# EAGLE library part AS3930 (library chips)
Single Channel Low Frequency Wakeup Receiver
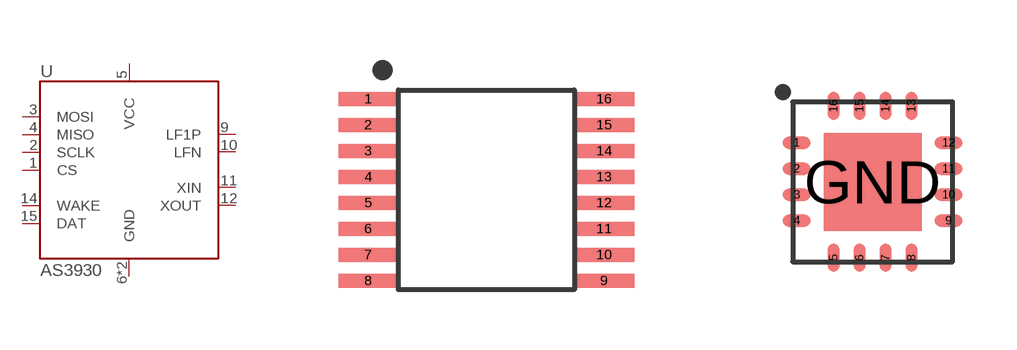
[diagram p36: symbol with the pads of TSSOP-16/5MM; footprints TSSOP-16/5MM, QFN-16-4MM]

Designator prefix U

## AS3930-BTST  [TSSOP-16/5MM]
1  CS
2  SCLK
3  MOSI
4  MISO
5  VCC
6  GND
9  LF1P
10  LFN
11  XIN
12  XOUT
13  GND
14  WAKE
15  DAT

## AS3930-BQFT (DIGIKEY: AS3930-BQFTCT-ND)  [QFN-16-4MM]
3  LF1P
4  LFN
5  XIN
6  XOUT
7  GND
8  WAKE
9  DAT
11  CS
12  SCLK
13  MOSI
14  MISO
15  VCC
16  GND
GND  GND

## Footprint TSSOP-16/5MM (pad centres in mm)
smd 1.5 x 0.35: 1 -2.95,2.275; 2 -2.95,1.625; 3 -2.95,0.975; 4 -2.95,0.325; 5 -2.95,-0.325; 6 -2.95,-0.975; 7 -2.95,-1.625; 8 -2.95,-2.275; 9 2.95,-2.275; 10 2.95,-1.625; 11 2.95,-0.975; 12 2.95,-0.325; 13 2.95,0.325; 14 2.95,0.975; 15 2.95,1.625; 16 2.95,2.275

## Footprint QFN-16-4MM (pad centres in mm)
smd 0.7 x 0.3: 1 -1.9,0.975; 2 -1.9,0.325; 3 -1.9,-0.325; 4 -1.9,-0.975; 9 1.9,-0.975; 10 1.9,-0.325; 11 1.9,0.325; 12 1.9,0.975
smd 0.3 x 0.7: 5 -0.975,-1.9; 6 -0.325,-1.9; 7 0.325,-1.9; 8 0.975,-1.9; 13 0.975,1.9; 14 0.325,1.9; 15 -0.325,1.9; 16 -0.975,1.9
smd 2.45 x 2.45: GND 0,0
